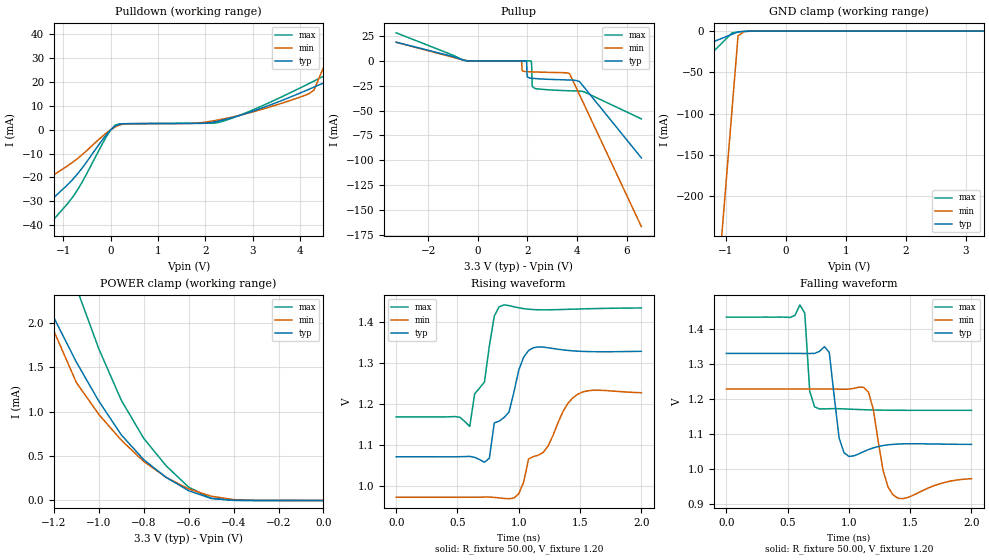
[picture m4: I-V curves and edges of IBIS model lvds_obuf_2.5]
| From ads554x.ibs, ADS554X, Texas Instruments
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|   Model lvds_obuf_2.5
[Model]   lvds_obuf_2.5
Model_type   3-state
Polarity   Non-Inverting
Enable   Active-High
Vmeas =   1.2000V
Cref =   5.0000pF
Rref = 50.0000
Vref =   1.2000V
C_comp   2.13pF   1.93pF   2.34pF
[Temperature Range]   27.00   125   -40.00
[Voltage Range]   3.30V   3.00V   3.60V
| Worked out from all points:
|   slope of the pulldown table from 0 to 0.495 V, typ, clamps not added: 190 ohm
|   GND clamp passes 1 mA (typ) near -0.79 V on its own axis
|   POWER clamp passes 1 mA (typ) near -0.97 V on its own axis
|   rising waveform, R_fixture 50.00, V_fixture 1.20: 20-80 % time 210ps typ, 303ps min, 143ps max; typ from 1.07 V to 1.33 V
|   falling waveform, R_fixture 50.00, V_fixture 1.20: 20-80 % time 51.2ps typ, 72.3ps min, 30ps max; typ from 1.33 V to 1.07 V
[Pulldown]
| voltage   I(typ)   I(min)   I(max)
-3.3V     -67.26mA   -46.2mA    -84.98mA
-2.1V     -45.06mA   -30.6mA    -57.86mA
-1.5V     -33.96mA   -22.8mA    -44.3mA
-800mV    -20.81mA   -13.61mA   -28.16mA
100mV     1.61mA     1.16mA     1.96mA
2.4V      4.17mA     4.57mA     3.7mA
4.3V      17.83mA    16.6mA     20.38mA
4.7V      21.47mA    35.52mA    24.41mA
4.9V      27.7mA     44.98mA    26.44mA
5.1V      46.62mA    54.44mA    28.67mA
5.5V      84.46mA    73.36mA    59.29mA
6.6V      188.5mA    125.4mA    177.8mA
[Pullup]
| voltage   I(typ)   I(min)   I(max)
-3.3V     18.96mA    18.87mA    28.4mA
-500mV    360uA      560uA      320uA
1.75V     21.45uA    9.44uA     40.53uA
1.79V     20.03uA    -9.718mA   38.18uA
1.95V     11.98uA    -10.68mA   28.76uA
1.99V     -15.56mA   -10.73mA   26.39uA
2.15V     -17.4mA    -10.91mA   7.593uA
2.17V     -17.45mA   -10.93mA   -4.721mA
2.2V      -17.51mA   -10.96mA   -25.88mA
3.7V      -19.14mA   -12.68mA   -30.04mA
4.1V      -20.69mA   -33.96mA   -30.36mA
6.6V      -97.69mA   -167mA     -58.36mA
[GND_clamp]
| voltage   I(typ)   I(min)   I(max)
-3.3V     -73.53mA   -2.228A    -176.7mA
-1.1V     -9.73mA    -272.6mA   -16.77mA
-1V       -6.83mA    -183.7mA   -9.5mA
-900mV    -3.93mA    -94.8mA    -2.23mA
-800mV    -1.03mA    -5.92mA    -1.19mA
-700mV    -450uA     -730uA     -490uA
3.3V      44.64pA    1.08uA     37.43pA
[POWER_clamp]
| voltage   I(typ)   I(min)   I(max)
-3.3V     247.8mA    491.9mA    558.7mA
-1.3V     2.62mA     3.21mA     3.99mA
-1.2V     2.06mA     1.91mA     3.16mA
-1.1V     1.56mA     1.33mA     2.4mA
-1V       1.12mA     970uA      1.71mA
-900mV    740uA      680uA      1.13mA
-800mV    460uA      440uA      700uA
-700mV    260uA      260uA      390uA
-600mV    110uA      130uA      150uA
-500mV    23.34uA    48.47uA    24.97uA
-400mV    2uA        9.55uA     1.31uA
0V        44.64pA    500pA      43.31pA
[Ramp]
| variable   typ   min   max
dV/dt_r   1.84/71.07p   1.61/0.12n   2.05/48.19p
dV/dt_f   1.31/99.15p   1.26/0.15n   1.37/67.18p
R_load = 1.00k
[Rising Waveform]
R_fixture = 50.00
V_fixture = 1.20
V_fixture_min = 1.10
V_fixture_max = 1.30
| time   V(typ)   V(min)   V(max)
0s        1.071V     971.9mV    1.168V
600ps     1.072V     972mV      1.145V
760ps     1.067V     972.3mV    1.341V
800ps     1.153V     971.6mV    1.414V
840ps     1.157V     970.3mV    1.437V
920ps     1.18V      968.4mV    1.439V
1ns       1.282V     980.4mV    1.434V
1.12ns    1.337V     1.071V     1.429V
1.48ns    1.328V     1.223V     1.431V
2ns       1.328V     1.227V     1.433V
[Falling Waveform]
R_fixture = 50.00
V_fixture = 1.20
V_fixture_min = 1.10
V_fixture_max = 1.30
| time   V(typ)   V(min)   V(max)
0s        1.33V      1.228V     1.433V
600ps     1.33V      1.228V     1.468V
640ps     1.329V     1.228V     1.444V
680ps     1.33V      1.228V     1.223V
800ps     1.349V     1.228V     1.172V
920ps     1.089V     1.228V     1.172V
1ns       1.037V     1.228V     1.171V
1.16ns    1.056V     1.219V     1.169V
1.36ns    1.071V     927.2mV    1.168V
2ns       1.071V     973.4mV    1.168V
